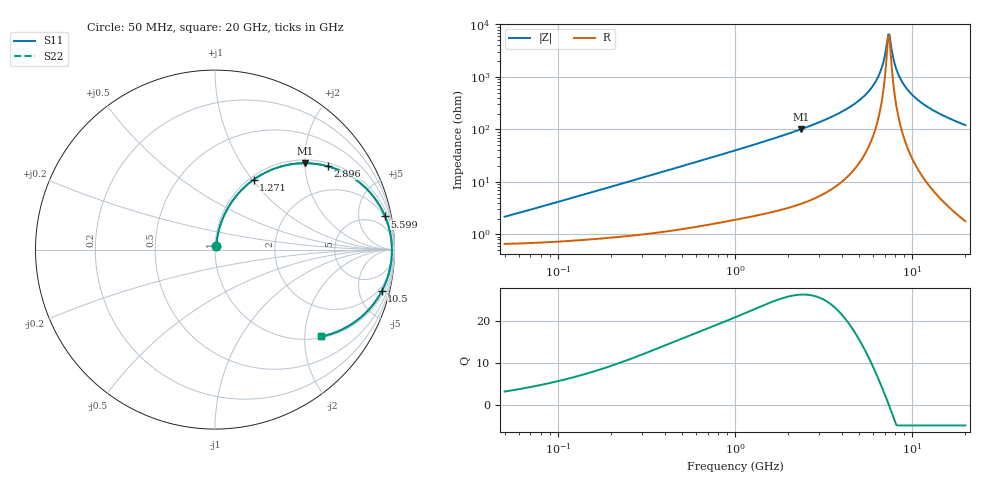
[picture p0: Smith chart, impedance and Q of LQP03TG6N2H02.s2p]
!Murata Part Number: LQP03TG6N2H02
!These Parameters are Measured in Series Mode Connection
!  o--[Z]--o
!Port1  Port2
!  o-------o
!Freq. Start=50[MHz] Stop=20[GHz], 401[Steps]
# Hz S RI R 50
!Freq.(Hz) S11(Real) S11(Imag) S21(Real) S21(Imag) S12(Real) S12(Imag) S22(Real) S22(Imag)
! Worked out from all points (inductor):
!   401 points, 50 MHz to 20 GHz, reference 50 ohm
!   read as one part in series: L = 6.57 nH near 51.52 MHz
!   highest Q = 26.4 at 2.349 GHz (marker M1), where L = 6.81 nH
!   self-resonance near 7.331 GHz
!   S11 on the Smith chart (normalised r, x): 50 MHz: 1.01, +0.04; 1.271 GHz: 1.04, +1.02; 2.896 GHz: 1.10, +2.63; 5.599 GHz: 2, +10; 10.5 GHz: 1.41, -7.85; 20 GHz: 1.04, -2.42
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5e7  0.00696 0.0204  0.993 -0.0204  0.993 -0.0204  0.00696 0.0204
1.364002e8  0.0107 0.0545  0.9893 -0.0545  0.9893 -0.0545  0.0107 0.0545
3.721004e8  0.0317 0.1423  0.9683 -0.1423  0.9683 -0.1423  0.0317 0.1423
1e9  0.148 0.332  0.852 -0.332  0.852 -0.332  0.148 0.332
1.270815e9  0.2155 0.3899  0.7845 -0.3899  0.7845 -0.3899  0.2155 0.3899
2.348516e9  0.5025 0.4814  0.4975 -0.4814  0.4975 -0.4814  0.5025 0.4814
2.728004e9  0.5922 0.4727  0.4078 -0.4727  0.4078 -0.4727  0.5922 0.4727
2.896447e9  0.6286 0.4643  0.3714 -0.4643  0.3714 -0.4643  0.6286 0.4643
4.275624e9  0.8465 0.3365  0.1535 -0.3365  0.1535 -0.3365  0.8465 0.3365
5.598765e9  0.9475 0.1849  0.0525 -0.1849  0.0525 -0.1849  0.9475 0.1849
6.125241e9  0.9677 0.1268  0.0323 -0.1268  0.0323 -0.1268  0.9677 0.1268
6.503449e9  0.9771 0.0869  0.0229 -0.0869  0.0229 -0.0869  0.9771 0.0869
6.802353e9  0.9818 0.0564  0.0182 -0.0564  0.0182 -0.0564  0.9818 0.0564
7.222371e9  0.9852 0.0155  0.0148 -0.0155  0.0148 -0.0155  0.9852 0.0155
7.442007e9  0.9856 -0.00508  0.0144 0.00508  0.0144 0.00508  0.9856 -0.00508
7.554318e9  0.9855 -0.0154  0.0145 0.0154  0.0145 0.0154  0.9855 -0.0154
8.020766e9  0.9828 -0.0564  0.0172 0.0564  0.0172 0.0564  0.9828 -0.0564
8.516016e9  0.9766 -0.0972  0.0234 0.0972  0.0234 0.0972  0.9766 -0.0972
9.316812e9  0.961 -0.157  0.039 0.157  0.039 0.157  0.961 -0.157
1.050288e10  0.9286 -0.2328  0.0714 0.2328  0.0714 0.2328  0.9286 -0.2328
1.375312e10  0.8135 -0.3763  0.1865 0.3763  0.1865 0.3763  0.8135 -0.3763
2e10  0.5926 -0.4841  0.4074 0.4841  0.4074 0.4841  0.5926 -0.4841
